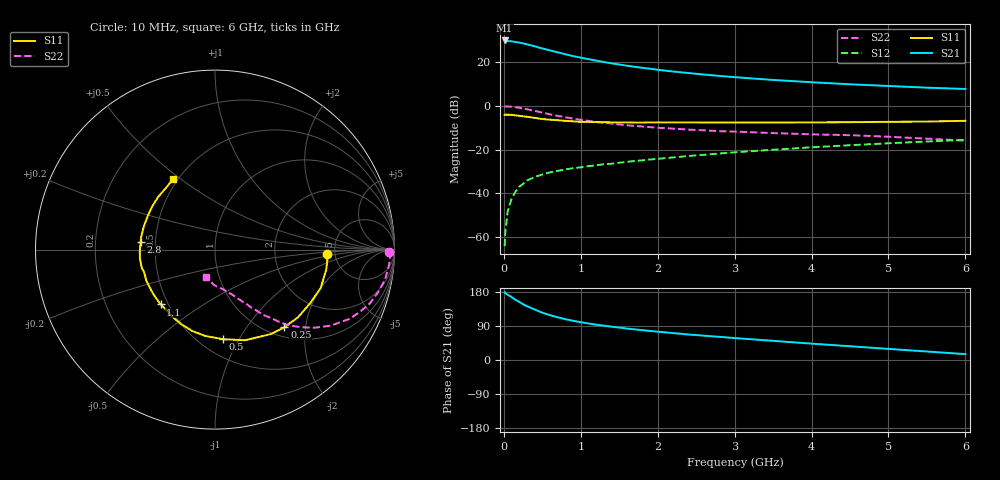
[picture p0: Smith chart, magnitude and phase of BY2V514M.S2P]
! SIEMENS Small Signal Semiconductors
! BFY420
! Si NPN RF SIEGET Grounded Emitter Transistor in MICRO-X
! VCE = 2.5 V  IC = 14 mA
! Common Emitter S-Parameters:  October  1996
# GHz  S  MA  R  50
!  f  S11  S21  S12  S22
! GHz  MAG  ANG  MAG  ANG  MAG  ANG  MAG  ANG
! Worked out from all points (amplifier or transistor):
!   36 points, 10 MHz to 6 GHz, reference 50 ohm
!   highest |S21| = 30.1 dB at 10 MHz (marker M1)
!   |S21| within 3 dB of that: start of sweep to 432.8 MHz
!   unconditionally stable (mu >= 1): 2.25 GHz to end of sweep
!   at 250 MHz: K = 0.24, MSG = 32.3 dB, |S12| = -35.8 dB
!   at 1.4 GHz: K = 0.84, MSG = 23.1 dB, |S12| = -26.5 dB
!   at 6 GHz: K = 1.08, MAG = 9.9 dB, |S12| = -15.6 dB
!   S11 on the Smith chart (normalised r, x): 10 MHz: 4.34, -0.33; 250 MHz: 1.18, -1.53; 500 MHz: 0.65, -0.86; 1.1 GHz: 0.45, -0.34; 2.8 GHz: 0.41, +0.04; 6 GHz: 0.47, +0.47
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0.01  0.6272 -2.1  32.08 178.8  0.0006 99.3  0.9717 -0.7
0.02  0.629 -4.3  31.96 176.1  0.0013 83.3  0.9775 -1.7
0.05  0.6296 -10.3  31.06 172.2  0.0038 87.7  0.9741 -4.9
0.1  0.6266 -20.0  30.64 166.3  0.0073 79.6  0.9618 -10.1
0.15  0.6082 -29.6  29.58 158.8  0.0107 75.6  0.9377 -14.9
0.2  0.5967 -39.3  28.7 153.4  0.0139 73.2  0.9124 -19.3
0.25  0.5797 -48.2  27.49 147.1  0.0162 69.5  0.8767 -23.5
0.3  0.5654 -56.2  26.16 142.0  0.0193 67.5  0.8437 -27.2
0.4  0.5323 -71.6  23.6 133.2  0.0233 62.8  0.7705 -33.4
0.5  0.5012 -84.8  21 124.7  0.0266 60.0  0.7027 -38.3
0.7  0.471 -105.6  17.13 112.6  0.0323 56.1  0.594 -45.4
0.8  0.456 -114.5  15.44 107.7  0.0347 53.4  0.5492 -47.9
0.9  0.4442 -121.4  14.04 103.4  0.0373 53.8  0.5131 -49.6
1.1  0.4303 -134.8  11.95 96.3  0.0415 53.5  0.4554 -53.3
1.3  0.424 -144.0  10.25 90.5  0.0459 53.0  0.4107 -55.7
1.6  0.4198 -156.3  8.418 82.9  0.052 52.9  0.3608 -59.2
2.2  0.421 -173.1  6.196 71.0  0.0657 52.0  0.3024 -64.9
2.8  0.4168 174.2  4.923 61.1  0.0808 50.0  0.2635 -69.8
3.5  0.4174 161.3  3.967 50.6  0.0988 46.3  0.2384 -75.4
4.5  0.4247 145.3  3.153 36.3  0.1254 39.3  0.2133 -84.2
5.5  0.4388 128.6  2.638 22.4  0.1528 30.7  0.1773 -98.3
6  0.4563 121.0  2.461 15.5  0.1659 26.1  0.1603 -108.1
